(* Logix 5000 Rung export; software revision 16.04 *)

MODULES
   Local : vendor None type None code None
   MVI56E_AFC : vendor None type None code None
END_MODULES

TYPE AFCEProveProcess :   // Prove process output from processor to the module
STRUCT
   Sequencing : AFCEProveSequencing;   // Prover sequencing
   Temperature : REAL;   // Temperature for Single Probe provers. And Inlet Temperature for Dual Probe Provers.
   OutletTemperature : REAL;   // Outlet Temperature for Provers with Dual Probes.
   SwitchBarTemperature : REAL;   // Switch bar temperature
   Pressure : REAL;   // Pressure for Single Probe provers. And Inlet Pressure for Dual Probe Provers.
   OutletPressure : REAL;   // Outlet Pressure for Provers with Dual Probes.
   ProverDensity : REAL;   // Prover density
END_STRUCT
END_TYPE

TYPE AFCEMeterControl :   // Enable/Disable Meter and Streams
STRUCT
   Meter : AFCEMeterControlMeter;   // Control the Meter
   Stream : AFCEMeterControlStream;   // Control the Meter Streams
   ResetAccumulators : AFCEMeterSignals;   // Resets for meter accumulators
END_STRUCT
END_TYPE

TYPE AFCEModbusMasterDataType :   // Modbus master data type
STRUCT
   Bit : BOOL;   // bit type
   Word : BOOL;   // word type (16-bit)
   Long : BOOL;   // long integer (32-bit)
   LongRemote : BOOL;   // long integer (32-bit)
END_STRUCT
END_TYPE

TYPE AFCEProveSequencing :   // AFC prove sequencing tag for phase selection and ball positioning
STRUCT
   Phase : AFCEProvePhaseBitmap;   // AFC phase sequencing
   BallPositionReady : BOOL;   // Ball position: Ready (Udir & Bdir only; fwd leg Bdir)
   BallPositionSealed : BOOL;   // Ball position: Sealed (Udir & Bdir only; fwd leg Bdir)
   BallPositionReadyBwdLeg : BOOL;   // Ball position: Ready bwd leg (Bdir only)
   BallPositionSealedBwdLeg : BOOL;   // Ball position: Sealed bwd leg (Bdir only)
END_STRUCT
END_TYPE

TYPE AFCEMeterLinearLiquidArchiveWrite :   // Write Archive
STRUCT
   Daily : BOOL;   // Set to 1 to write daily archive
   Hourly : BOOL;   // Set to 1 to write hourly archive
END_STRUCT
END_TYPE

TYPE AFCEMeterLinearLiquidProcess :   // Linear Liquid Process Variables
STRUCT
   PulseFrequency : REAL;   // Pulse frequency (Hz)
   Temperature : REAL;   // Temperature
   Pressure : REAL;   // Pressure
   Density : REAL;   // Density
   WaterPercent : REAL;   // Water (%)
   MeterPulses : DINT;   // Meter pulses
END_STRUCT
END_TYPE

TYPE AFCEMeterLinearLiquidAlarm :
STRUCT
   Control : AFCEMeterLinearLiquidAlarmControl;   // Alarm Control
END_STRUCT
END_TYPE

TYPE AFCEUtil :   // Used for internal ladder logic usage. These values must not be changed by user application.
STRUCT
   Flags : AFCEFlag;   // Wallclock update commands
   CycleCounter : INT;   // Reflects current block ID calculated by ladder to be sent to the module
   Buffer : AFCEUtilBuffer;
   Block : AFCEUtilBlock;
END_STRUCT
END_TYPE

TYPE AFCEExtended :
STRUCT
   Trigger : BOOL;
   Data : AFCEExtendedData;
END_STRUCT
END_TYPE

TYPE AFCEModbusGatewayCommand :   // Modbus Gateway Command
STRUCT
   Config : AFCEModbusGatewayConfig;   // Config data to be entered by the user.
   Trigger : BOOL;   // Trigger the Command, when cleared module has responded.
   Data : INT[200];   // Contains modbus data written to the module (write commands)
END_STRUCT
END_TYPE

TYPE AFCEMeterLinearLiqBackPlaneReturn :   // Linear Liquid Meter
STRUCT
   StandardDefault : AFCEMeterLinearLiquidStandardDflt;
   StandardRaw : INT[14];
   Extended : AFCEExtended;
END_STRUCT
END_TYPE

TYPE AFCEMeterStatusStream :
STRUCT
   Active : INT;   // Current Active Stream
   Enabled : AFCEMeterStatusStreamEnabled;   // Enabled Streams
   Configured : AFCEMeterStatusStreamEnabled;   // Configured Streams
   EnableAlarm : AFCEMeterStatusStreamAlarm;   // Enable Alarms
END_STRUCT
END_TYPE

TYPE AFCEProveRunResults :   // Run results of the prove. Copied from the module to the pocessor
STRUCT
   CountAttempted : INT;   // Run count attempted
   CountCompleted : INT;   // Run count completed
   CountSelected : INT;   // Run count selected
   RunsSelected : INT;   // Bit Mapped Runs selected for calculations from completed runs
   NewMeterFactor : REAL;   // New meter factor
   ChangeInMeterFactor : REAL;   // Change in meter factor
END_STRUCT
END_TYPE

TYPE AFCEModbusMasterSwap :   // Modbus master swap words/ swap bytes
STRUCT
   SwapWords : BOOL;   // Swap words
   SwapBytes : BOOL;   // Swap bytes
END_STRUCT
END_TYPE

TYPE AFCEModbusMaster :   // Modbus Master. Port 3 must be configured as modbus master through AFC Manager to use this feature.
STRUCT
   Enable : BOOL;   // Enable the modbus master funcionality
   CommandIndex : INT;   // Selects which command index will be executed
   Command : AFCEModbusMasterCommand[10];   // Each command contains a specific modbus request to be sent out of the port
END_STRUCT
END_TYPE

TYPE AFCEMeterLinearLiquidCalRequestProces :
STRUCT
   PulseFrequency : BOOL;   // Pulse Frequency
   Temperature : BOOL;   // Temperature
   Pressure : BOOL;   // Pressure
   Density : BOOL;   // Density
   WaterContent : BOOL;   // Water Content
END_STRUCT
END_TYPE

TYPE AFCEFlag :   // Flags contains status information updated by ladder and also trigger bits for clock update
STRUCT
   AFCStopped : BOOL;   // Indicates that the module has sent a new input block to be processed by ladder - UPDATED BY LADDER
   AFCInputSequenceNum : INT;   // Meter number (0 -15) associated to blocks 1-16. Used to update "Profile" (meter type and product group.) UPDATED BY LADDER
END_STRUCT
END_TYPE

TYPE AFCEModbusPassThruBitData :   // AFC Modbus Pass-thru Bit Data
STRUCT
   Data : BOOL[2016];   // Contains received data for bit commands
END_STRUCT
END_TYPE

TYPE AFCEUtilBlockInterrupt :
STRUCT
   Now : BOOL;
   ModbusGateway : DINT;
   EnableDisable : BOOL;
   Analysis : DINT;
END_STRUCT
END_TYPE

TYPE AFCEFirmwareVersion :
STRUCT
   Major : SINT;   // Major Version number
   Minor : SINT;   // Minor Version number
   Revision : INT;   // Revision
END_STRUCT
END_TYPE

TYPE AFCEModbusGateway :   // Modbus Gateway
STRUCT
   Command : AFCEModbusGatewayCommand[10];   // Modbus gateway commands - contains setup and modbus data
END_STRUCT
END_TYPE

TYPE AFCEMeterCalRequestActionType :
STRUCT
   ZeroShift : BOOL;   // Zero Shift
   SetZero : BOOL;   // Set Zero
   SetSpan : BOOL;   // Set Span
   SetMid1 : BOOL;   // Set Mid 1
   SetMid2 : BOOL;   // Set Mid 2
   SetMid3 : BOOL;   // Set Mid 3
END_STRUCT
END_TYPE

TYPE AFCEUtilBuffer :   // Buffer
STRUCT
   Input : INT[250];   // Input buffer contains the complete block to be copied from the module
   Output : INT[248];   // Output buffer contains data the complete block to be copied to the module
   Process : INT[240];
   ArchiveDay : INT[98];
   ArchiveHour : INT[98];
   Prove : INT[26];
   Analysis : INT[198];
   MeterEnableDisable : INT[4];
   StreamEnable : INT[48];
   StreamDisable : INT[48];
   StreamSelect : INT[32];
   MeterSignals : INT[32];
   Calibration : INT[36];
END_STRUCT
END_TYPE

TYPE AFCEUtilBlock :
STRUCT
   ProcessInput : INT;
   InterruptPending : AFCEUtilBlockInterrupt;
   InterruptComplete : AFCEUtilBlockInterrupt;
   NonInterruptPending : AFCEUtilBlockNonInterrupt;
   NonInterruptComplete : AFCEUtilBlockNonInterrupt;
END_STRUCT
END_TYPE

TYPE AFCEMeterSignals :   // Meter trigger accumulator and archive resets
STRUCT
   ResetAccumulator1 : BOOL;   // Set to 1 to reset resettable accumulator 1
   ResetAccumulator2 : BOOL;   // Set to 1 to reset resettable accumulator 2
   ResetAccumulator3 : BOOL;   // Set to 1 to reset resettable accumulator 3
   ResetAccumulator4 : BOOL;   // Set to 1 to reset resettable accumulator 4
END_STRUCT
END_TYPE

TYPE AFCEProve :   // Prove
STRUCT
   Process : AFCEProveProcess;   // Process Variables
   Signals : AFCEProveSignals;   // AFC Prove Signals (triggers the proving update)
   Config : AFCEProveConfig;   // AFC Prove Control (configuration settings)
   PulseCounts : AFCEProvePulseCount;   // Pulse counts to be updated at the end of the run/pass
   ConfigInput : AFCEProveInputConfig;   // AFC prover input configuration
   Status : AFCEProveStatus;   // AFC prover status
   ErrorCode : INT;   // Prove error code
   ProveControlsEcho : INT;   // AFC module Echos the state of the Prove Controls
   RequestedMeterEcho : INT;   // AFC module Echos the Meter number requested
   RequestedCurvePointEcho : INT;   // AFC module Echos the requested Curve Point
   RunResults : AFCEProveRunResults;   // Prove and run results
   ProveEnabled : BOOL;   // ON if prove is enabled. This flag is coped from inputbuffer[247]
END_STRUCT
END_TYPE

TYPE AFCEMeterControlStream :
STRUCT
   Selected : SINT;   // Stream to Enable or Disable and/or make active.
   EnableSelected : BOOL;   // Enable the Selected Stream
   DisableSelected : BOOL;   // Disable the Selected Stream
   SetSelectedToActive : BOOL;   // Set Selected to Active Stream
END_STRUCT
END_TYPE

TYPE AFCEProveConfig :   // Controls (configuration settings) associated to the prover
STRUCT
   Enable : AFCEProveConfigEnable;   // Controls at enable
   Accept : AFCEProveConfigAccept;   // Controls at accept
END_STRUCT
END_TYPE

TYPE AFCEWallclock :
STRUCT
   GetAFCTime : BOOL;   // Get current AFC Time
   SetAFCTimeFromPLCTime : BOOL;   // Set AFC time from PLC time. Updates current AFC time
   EnableLocalDateTime : BOOL;   // Enable Local Date Time.
   AFCTime : AFCETime;   // Coordinated Universal Time. Updated by either getting or setting AFC time.
END_STRUCT
END_TYPE

TYPE AFCEMeterCalRequestActionValue :
STRUCT
   ZeroShift : AFCEMeterCalRequestValue;   // Zero Shift
   SetZero : AFCEMeterCalRequestValue;   // Set Zero
   SetSpan : AFCEMeterCalRequestValue;   // Set Span
   SetMid1 : AFCEMeterCalRequestValue;   // Set Mid 1
   SetMid2 : AFCEMeterCalRequestValue;   // Set Mid 2
   SetMid3 : AFCEMeterCalRequestValue;   // Set Mid 3
END_STRUCT
END_TYPE

TYPE AFCEMeterStatus :   // Status
STRUCT
   Meter : AFCEMeterStatusMeter;   // Meter Status
   Stream : AFCEMeterStatusStream;   // Stream Status
END_STRUCT
END_TYPE

TYPE AFCEModbusMasterConfig :   // Modbus master command settings
STRUCT
   Enable : BOOL;   // Set to 1 to enable command (0=disable)
   FunctionType : BOOL;   // Set to 1 to select write command (0=read command)
   RegisterBank : BOOL;   // Set to 1 to select input register (0=holding register)
   DataType : AFCEModbusMasterDataType;   // Select data type format
   SwapOption : AFCEModbusMasterSwap;   // Select byte and word swap (1 = swap, 0 = no swap)
   TypeSwap : INT;   // This value is calculated by ladder logic and must not be modified by user
   SlaveAddress : INT;   // Modbus slave address of remote device
   ModbusAddress : INT;   // Modbus data address on remote slave
   ElementCount : INT;   // Number of data elements (125 words)
   TransactionID : INT;   // Transaction ID. This value is returned to the ReturnedTransaction ID when the response has been received.
END_STRUCT
END_TYPE

TYPE AFCEMeterStatusStreamEnabled :   // Stream Status 1 = Enabled
STRUCT
   Stream1 : BOOL;
   Stream2 : BOOL;
   Stream3 : BOOL;
   Stream4 : BOOL;
   Stream5 : BOOL;
   Stream6 : BOOL;
   Stream7 : BOOL;
   Stream8 : BOOL;
   Stream9 : BOOL;
   Stream10 : BOOL;
   Stream11 : BOOL;
   Stream12 : BOOL;
   Stream13 : BOOL;
   Stream14 : BOOL;
   Stream15 : BOOL;
   Stream16 : BOOL;
END_STRUCT
END_TYPE

TYPE AFCEMeterArchiveFetchError :
STRUCT
   ArchiveSelectionInvalid : BOOL;   // Archive File Selection Invalid
   AgeOutsideSize : BOOL;   // Age Outside Configured File Size
   ArchiveNeverWritten : BOOL;   // Age OK but Archive Record Never Written (new or reconfigured meter)
   Reserverd1 : BOOL;
   Reserverd2 : BOOL;
   Reserverd3 : BOOL;
   Reserverd4 : BOOL;
   Reserverd5 : BOOL;
   Reserverd6 : BOOL;
   Reserverd7 : BOOL;
   Reserverd8 : BOOL;
   Reserverd9 : BOOL;
   Reserverd10 : BOOL;
   Reserverd11 : BOOL;
   Reserverd12 : BOOL;
   Reserverd13 : BOOL;
END_STRUCT
END_TYPE

TYPE AFCEMeterLinearLiquidArchiveDflt :   // Default Configuration
STRUCT
   ClosingTimestamp : DINT;   // Closing Timestamp
   CumulativeActiveStreams : INT;
   CurrentActiveStream : SINT;
   MeterStatus : SINT;
   FlowingPeriod : DINT;
   PeriodDuration : DINT;
   AccumulatorTotalizer : DINT;
   AccumulatorResidue : REAL;
   MeterAlarms : DINT;
   PulseFrequency : REAL;
   Temperature : REAL;
   Pressure : REAL;
   Density : REAL;
   WaterContent : REAL;
   ReferenceDensity : REAL;
   Ctpl : REAL;
   KFactor : REAL;
   MeterFactor : REAL;
   InputPulseCount : DINT;
   ManPulseCountCurrent : DINT;
   MassNRAccumulatorCurrent : REAL;   // Non-resettable
   MassNRAccumulatorOpening : REAL;   // Non-resettable
   Available01 : INT;
   Available02 : INT;
   Available03 : INT;
   Available04 : INT;
   NetNRAccumulatorCurrent : REAL;   // Non-resettable
   NetNRAccumulatorOpening : REAL;   // Non-resettable
   GrossNRAccumulatorCurrent : REAL;   // Non-resettable
   GrossNRAccumulatorOpening : REAL;   // Non-resettable
   GrossStandardNRAccumulatorOpening : REAL;   // Non-resettable
   GrossStandardNRAccumulatorCurrent : REAL;   // Non-resettable
   WaterNRAccumulatorCurrent : REAL;   // Non-resettable
   WaterNRAccumulatorOpening : REAL;   // Non-resettable
   API2540VaporPressureAbsolute : REAL;
   Available05 : INT;
   Available06 : INT;
   UserSpecifiedFlowAverage1 : REAL;
   UserSpecifiedFlowAverage2 : REAL;
   UserSpecifiedFlowAverage3 : REAL;
END_STRUCT
END_TYPE

TYPE AFCEMeterLinearLiquidAlarmControl :   // Linear Liquid Process Alarms
STRUCT
   PulseFrequency : AFCEMeterProcessAlarm;   // Pulse Frequency Alarms
   Temperature : AFCEMeterProcessAlarm;   // Temperature Alarms
   Pressure : AFCEMeterProcessAlarm;   // Pressure Alarms
   Density : AFCEMeterProcessAlarm;   // Density Alarms
   WaterPercent : AFCEMeterProcessAlarm;   // Water Percent Alarms
   MeterPulses : AFCEMeterProcessAlarmFidelity;   // Meter Pulses Alarms
END_STRUCT
END_TYPE

TYPE AFCEMeterLinearLiquidCal :   // Processor Mediated Calibration
STRUCT
   Request : AFCEMeterLinearLiquidCalRequest;   // Calibration Request from module
   Response : AFCEMeterCalResponse;   // Processor Response
END_STRUCT
END_TYPE

TYPE AFCEMeterLinearLiquidArchive :   // Different Liquid Archive
STRUCT
   Write : AFCEMeterLinearLiquidArchiveWrite;
   Fetch : AFCEMeterLinearLiquidArchiveFetch;
END_STRUCT
END_TYPE

TYPE AFCESiteStatus :   // Site status bits - contains general information about the module - not meter specific
STRUCT
   AFCActive : BOOL;   // AFC active
   ChecksumAlarms : BOOL;   // Checkum alarm active
   Reserved2 : BOOL;
   Reserved3 : BOOL;
   PLCHalted : BOOL;   // PLC in program mode or missing
   CfgChanged : BOOL;   // Configuration changed
   Powerup : BOOL;   // Module powered up
   ColdStart : BOOL;   // Module performed cold start (BBRAM initialized)
   ModbusMasterPending : BOOL;   // Modbus Master Poll Pending
   ModbusMasterComplete : BOOL;   // Modbus Master Poll Complete
   ModbusPassThruPending : BOOL;   // Modbus Pass-thru Input Pending
   CalibrationRequest : BOOL;   // Calibration request from module
   ProverEnabled : BOOL;   // Prover Enabled
   Reserved13 : BOOL;
   Reserved14 : BOOL;
   Reserved15 : BOOL;
END_STRUCT
END_TYPE

TYPE AFCEModuleDef :   // Main user defined data type
STRUCT
   ModbusGateway : AFCEModbusGateway;   // Reads and write data between processor and module modbus table
   ModbusMaster : AFCEModbusMaster;   // Setup modbus master commands to be sent to remote slaves (through Port 3)
   ModbusPassThru : AFCEModbusPassThru;   // Modbus pass-thru data
   SiteStatus : AFCESiteStatus;   // Site status
   MeterAlarms : AFCESiteAlarms;   // Meter Alarms
   Prove : AFCEProve;   // Prover
   Wallclock : AFCEWallclock;   // Set clock and get clock information
   Firmware : AFCEFirmwareVersion;   // Firmware information
   Util : AFCEUtil;   // Used by ladder logic
END_STRUCT
END_TYPE

TYPE AFCEModbusGatewayConfig :   // Modbus Ggateway Configuration
STRUCT
   Enable : BOOL;   // Set to 1 to enable modbus gateway command (0=disable)
   StartRegister : DINT;   // Start modbus address
   RegisterCount : INT;   // Word count (200 max)
   FunctionType : BOOL;   // 0 = read command, 1 = write command
   RegisterType : BOOL;   // 0 = holding register, 1 = input register
   SlaveType : BOOL;   // 0 = primary slave, 1 = virtual slave
END_STRUCT
END_TYPE

TYPE AFCEMeterLinearLiquidArchiveFetchT :   // Fetch Archive
STRUCT
   Trigger : BOOL;   // Trigger Archive Fetch
   Age : INT;   // 0 = Current Archive
   Error : AFCEMeterArchiveFetchError;   // Archive Fetch Error
   Default : AFCEMeterLinearLiquidArchiveDflt;   // Default Archive
   Raw : INT[100];   // Raw Archive
END_STRUCT
END_TYPE

TYPE AFCEMeterCalRequestValue :
STRUCT
   Applied : REAL;   // Applied
   Measured : REAL;   // Measured
END_STRUCT
END_TYPE

TYPE AFCEMeterProcessAlarmFidelity :   // Process Alarms
STRUCT
   SetGeneralFail : BOOL;   // Set to indicate General Failure of the Transmitter
   StaleData : BOOL;   // Clear to Indicate new process input data
   Reserved : BOOL;   // Reserved
   SetPulseFidelityAlarm : BOOL;   // Set to indicate Pulse Fidelity Alarm
   SetAutoClearStaleData : BOOL;   // Set to automatically clear stale data
END_STRUCT
END_TYPE

TYPE AFCEUtilBlockNonInterrupt :
STRUCT
   Now : BOOL;
   ModbusMasterCommand : BOOL;
   ModbusMasterResponse : BOOL;
   Archive : DINT;
   Prover : BOOL;
   PassThru : BOOL;
   Calibration : BOOL;
END_STRUCT
END_TYPE

TYPE AFCEMeterLinearLiquid :   // Linear Liquid Meter
STRUCT
   Control : AFCEMeterControl;   // Meter Control
   Status : AFCEMeterStatus;   // Meter Status
   ProcessVariables : AFCEMeterLinearLiquidProcess;   // Input process variables to be transferred to the module
   Alarm : AFCEMeterLinearLiquidAlarm;   // Meter Alarms
   Archive : AFCEMeterLinearLiquidArchive;   // Archive
   Profile : AFCEMeterProfile;   // Module profile (meter type/product group) transfered from the module
   Calibration : AFCEMeterLinearLiquidCal;   // Calibration
   BackPlaneReturn : AFCEMeterLinearLiqBackPlaneReturn;
END_STRUCT
END_TYPE

TYPE AFCEProveConfigAccept :   // Prove controls at accept. If auto-accept is selected must be available at enable
STRUCT
   RequestedInterpolationPoint : INT;   // Requested interpolation point (0 nearest)
   ApplyMFChangeAllStreams : BOOL;   // Apply change in meter factor to all streams
   ApplyMFChangeCurve : BOOL;   // Apply change in meter factor to all curve points
   ApplyNewMF : BOOL;   // CApply new meter factor
END_STRUCT
END_TYPE

TYPE AFCEProvePhaseBitmap :   // AFC prove phase bitmap
STRUCT
   NotSelected : BOOL;   // Not selected
   Active : BOOL;   // Active, not counting
   CountingPast1stSwitch : BOOL;   // Counting past 1st switch for Udir and forward leg for Bdir)
   Past2ndSwitchFwdLeg : BOOL;   // Past 2nd switch forward leg (bidirectional only)
   Past1stSwithRetLeg : BOOL;   // Past 1st switch return leg (bidirectional only)
   RunComplete : BOOL;   // Run complete. past 2nd switch.
END_STRUCT
END_TYPE

TYPE AFCETime :   // AFC time format used for wallclock update.
STRUCT
   Year : DINT;   // Year
   Month : DINT;   // Month
   Day : DINT;   // Day
   Hour : DINT;   // Hour
   Minute : DINT;   // Minute
   second : DINT;   // Seconds
END_STRUCT
END_TYPE

TYPE AFCEProveSignals :   // Contains the proving signals that will trigger specific tasks from the module
STRUCT
   EnableProve : BOOL;   // Enables the prove
   AcceptProve : BOOL;   // Accepts the prove
   RejectProve : BOOL;   // Reject the prove
   RunStart : BOOL;   // Starts the run
   RunComplete : BOOL;   // Flags that the run is complete
   RunCancel : BOOL;   // Cancels the run
   RunDelete : BOOL;   // Deletes the run
   PassComplete : BOOL;   // Flag that the pass is complete
   PauseProve : BOOL;   // Pauses the Proving Process
   AbortProve : BOOL;   // Aborts the prove
END_STRUCT
END_TYPE

TYPE AFCEMeterProfile :   // Meter configuration profile
STRUCT
   MeterType : BOOL;   // 0=Differential, 1=Linear
   ProductGroup : BOOL;   // 0=Gas, 1=Liquid
   PrimaryInput : BOOL;   // For differential, 0=Differential Pressure 1=Flow Rate. For Linear, 0=Pulse Count 1=Pulse Frequency
   AOIMismatch : BOOL;   // AOI Meter type does not match module for meter number
END_STRUCT
END_TYPE

TYPE AFCEMeterStatusStreamAlarm :   // Stream Alarms
STRUCT
   StreamOutOfRange : BOOL;   // Requested Stream Number Out of Range
   StreamNotConfigured : BOOL;   // Requested Stream not Configured
   StreamNotEnabled : BOOL;   // Requested Stream not Enabled
   EventLogFull : BOOL;   // Event Log Full, Action not Performed
END_STRUCT
END_TYPE

TYPE AFCEModbusPassThru :   // AFC Modbus Pass-thru
STRUCT
   Enable : BOOL;   // Set to 1 to enable pass-thru functionality (requires AFC Manager setting)
   MessagePresent : BOOL;   // Message present in the response block
   GetMessage : BOOL;   // Get the pass-thru message. When the bit is cleared the message has been transferred to the PLC.
   FunctionBitWrite : BOOL;   // Function bit write
   OverflowError : BOOL;   // Overflow error flag
   ModbusAddress : INT;   // Destination modbus address
   RegisterCount : INT;   // Number of elements associated to command
   ReadDataWord : INT[125];   // Contains received data for word commands
   ReadDataBit : AFCEModbusPassThruBitData;   // Contains received data for bit commands
END_STRUCT
END_TYPE

TYPE AFCEProveInputConfig :   // Prove input block results - prover configuration
STRUCT
   Type : INT;   // Prover type
   Options : INT;   // Prover options
   RunsPerProveTotal : INT;   // Total runs per prove
   RunsPerProveSelected : INT;   // Selected runs per prove
   MaxRunsBeforeAbort : INT;   // Max total runs before abort
   ShortPassesPerRun : INT;   // Short passes per run if bidir = 2 , else 0
END_STRUCT
END_TYPE

TYPE AFCEMeterLinearLiquidArchiveFetch :
STRUCT
   Daily : AFCEMeterLinearLiquidArchiveFetchT;
   Hourly : AFCEMeterLinearLiquidArchiveFetchT;
END_STRUCT
END_TYPE

TYPE AFCEMeterLinearLiquidStandardDflt :   // Linear Liquid Meter Default Standard Data
STRUCT
   Meter_Alarms : DINT;   // Meter alarms
   NR_Acc_Net_Totalizer : DINT;   // Non-resettable accumulator, net, totalizer (m3)
   NR_Acc_Net_Residue : REAL;   // Non-resettable accumulator, net, residue (m3)
   FlowRate_Net : REAL;   // Flow rate, net (m3/h)
   NR_Acc_Gross_Totalizer : DINT;   // Non-resettable accumulator, gross / indicated, totalizer (m3)
   NR_Acc_GrossStandard_Totalizer : DINT;   // Non-resettable accumulator, gross standard, totalizer (m3)
   NR_Acc_Mass_Totalizer : DINT;   // Non-resettable accumulator, mass, totalizer (kg)
END_STRUCT
END_TYPE

TYPE AFCEProveStatus :   // Status of the prove (returned from the module to the processor)
STRUCT
   ProveAccepted : BOOL;   // Prove was accepted
   MeterFactorApplied : BOOL;   // Meter factor was applied
   MFAppliedToCurve : BOOL;   // Meter factor was applied to all points in the curve
   MFAppliedToStreams : BOOL;   // Meter factor was applied to all streams
   ProveRejectedByCommand : BOOL;   // Prove was rejected by command
   ProveRejectedNoRuns : BOOL;   // Prove was rejected - empty prove (no runs)
   ProveRejectedDivideBy0 : BOOL;   // Prove was rejected - divide by 0
   ProveEnabled : BOOL;   // Prove is enabled
   ProvingRunInProgress : BOOL;   // Proving run is in progress
   ProveRejectedAbort : BOOL;   // Prove rejected: abort
   ProvePaused : BOOL;   // Prove is paused
   RunCancelled : BOOL;   // Run Is cancelled
   RunTimedOut : BOOL;   // Run timed out
END_STRUCT
END_TYPE

TYPE AFCEMeterProcessAlarm :   // Process Alarms
STRUCT
   SetGeneralFail : BOOL;   // Set to indicate General Failure of the Transmitter
   StaleData : BOOL;   // Clear to Indicate new process input data
   SetLowThreshold : BOOL;   // Set to indicate Lower Range Limit Exceeded
   SetHighThreshold : BOOL;   // Set to indicate Upper Range Limit Exceeded
   SetAutoClearStaleData : BOOL;   // Set to automatically clear stale data
END_STRUCT
END_TYPE

TYPE AFCEProveConfigEnable :   // Prove controls at enable
STRUCT
   MeterNumber : INT;   // Meter number requested (1-16)
   AutoAcceptProve : BOOL;   // Auto-accept the prove
   AutoContinueProve : BOOL;   // Auto-continue the prove
END_STRUCT
END_TYPE

TYPE AFCEMeterStatusMeter :   // Meter Status
STRUCT
   Enabled : BOOL;   // Meter Enable Status, 1=enabled
   EnableAlarm : BOOL;   // If set either: 1. The meter is not configured. 2. The event log is full, the action was not performed.
END_STRUCT
END_TYPE

TYPE AFCEMeterControlMeter :   // Enable and Disable Meter
STRUCT
   Enable : BOOL;   // Enable the Meter
   Disable : BOOL;   // Disable the Meter
END_STRUCT
END_TYPE

TYPE AFCEModbusMasterCommand :   // Modbus Master Command
STRUCT
   Config : AFCEModbusMasterConfig;   // Modbus Master Configuration
   ErrorCode : INT;   // Error Code associated to Modbus Master Command
   Pending : BOOL;   // Pending Modbus Master Command - waiting for Modbus Response
   ReturnedTransactionID : DINT;   // Changes to Config.TransactionID value when response has returned.
   Data : INT[100];   // Read or Write Data
END_STRUCT
END_TYPE

TYPE AFCEProvePulseCount :   // Values to be supplied at the end of the pass/run
STRUCT
   Meter : DINT;   // Meter pulse count
   MasterMeter : DINT;   // Master meter pulse count
END_STRUCT
END_TYPE

TYPE AFCEMeterCalResponse :
STRUCT
   Trigger : BOOL;   // Send Error Code and Values to module to be recorded
   ErrorCode : SINT;   // Error Code to send. 0-4 allowed. 0=No error. 1-4=User defined.
   Value : AFCEMeterCalRequestValue;   // Value to Send
   Count : DINT;   // Number of calibration responses
END_STRUCT
END_TYPE

TYPE AFCEExtendedData :
STRUCT
   Raw : INT[64];
END_STRUCT
END_TYPE

TYPE AFCEMeterLinearLiquidCalRequest :
STRUCT
   ProcessVariable : AFCEMeterLinearLiquidCalRequestProces;   // Process Variable
   ActionType : AFCEMeterCalRequestActionType;   // Action Type
   Value : AFCEMeterCalRequestActionValue;   // Value
   Count : DINT;   // Number of calibration requests
END_STRUCT
END_TYPE

TYPE AFCESiteAlarms :   // Indicates if a meter has any alarms
STRUCT
   Meter1 : BOOL;   // Meter in alarm
   Meter2 : BOOL;   // Meter in alarm
   Meter3 : BOOL;   // Meter in alarm
   Meter4 : BOOL;   // Meter in alarm
   Meter5 : BOOL;   // Meter in alarm
   Meter6 : BOOL;   // Meter in alarm
   Meter7 : BOOL;   // Meter in alarm
   Meter8 : BOOL;   // Meter in alarm
   Meter9 : BOOL;   // Meter in alarm
   Meter10 : BOOL;   // Meter in alarm
   Meter11 : BOOL;   // Meter in alarm
   Meter12 : BOOL;   // Meter in alarm
   Meter13 : BOOL;   // Meter in alarm
   Meter14 : BOOL;   // Meter in alarm
   Meter15 : BOOL;   // Meter in alarm
   Meter16 : BOOL;   // Meter in alarm
END_STRUCT
END_TYPE

ADD_ON_INSTRUCTION AOI56EAFCMeterLinearLiquid   (* revision 1.7, vendor ProSoft Technology Inc., ExecutePrescan *)
// Add-On instruction for the MVI56E-AFC.
// Linear Liquid Meter
// Revision note:
// Corrected/Reverted ProcessInputBlockID Tag Data Type from INT to DINT.
// Help:
// v1.3: Addition of default process input backplane return data mapping.
// v1.4: Made correlation changes between the Module Archive Default UDTs and the AOI Archive Default UDTs.
// v1.5:  Made changes to the ModbusGatewayConfig UDT StartRegister Tag Data Type from INT to DINT
// and Modified ProcessInputBlockID Tag Data Type from DINT to INT.
// v1.6:  Updated Tags names AFCMeterXXYYYYYY.BackPlaneReturn.ProcessInputs to
// AFCMeterXXYYYYYY.BackPlaneReturn.Standard and
// AFCMeterXXYYYYYY.BackPlaneReturn.ComponentAnalysis
//  to AFCMeterXXYYYYYY.BackPlaneReturn.Extended.
// v1.7:  Corrected/Reverted ProcessInputBlockID Tag Data Type from INT to DINT.
VAR_IN_OUT
   ConnectionInput : INT[250]; {required}
   AFC : AFCEModuleDef; {required}
   AFCMeter : AFCEMeterLinearLiquid; {required}
END_VAR
VAR_INPUT
   MeterNumber : SINT; {required}   // Meter Number Set to a number between 1 and 16
END_VAR
VAR
   StreamSelectedShift : DINT;
   StreamSelectBuffer : INT;
   EnabledStatusBuffer : INT;
   StreamSelectBlockID : DINT;
   StreamNumberShift : DINT;
   StreamErrorBuffer : DINT;
   StreamEnableBlockID : DINT;
   StreamEnableBitPosition : DINT;
   StreamDisableBlockID : DINT;
   ResetOnce : BOOL;
   ProfileBuffer : SINT[2];
   ProcessInputBlockID : DINT;
   AnalysisGroupBitPosition : INT;
   AnalysisErrorBuffer : INT;
   ProcessAlarmShifter : DINT;
   ProcessAlarmHolder : DINT;
   ProcessAlarmBuffer : DINT;
   MeterSignaltBlockID : DINT;
   MeterNumberShift : DINT;
   MeterNumberBitPostition : DINT;
   Inputbuffer : INT[250];
   CalibrationMeterNumberBuffer : DINT;
   CalibrationMediationPending : BOOL;
   CalibrationInputScalingIndex : DINT;
   CalibrationHandleBuffer : DINT;
   ArchiveStream : DINT;
   ArchiveMeterStatusRaw : DINT;
   ArchiveMeterStatusActiveStream : DINT;
   ArchiveCompleteBitCheck : DINT;
   ArchiveBlockID : DINT;
   AnalysisGroupShift : DINT;
   AnalysisCompleteBitCheck : DINT;
   AnalysisBufferOffset : DINT;
   AFCStopped : BOOL;
   AFCInputDataAvailable : BOOL;
   AnalysisBlockID : DINT;
END_VAR

ROUTINE Logic   (* ladder *)
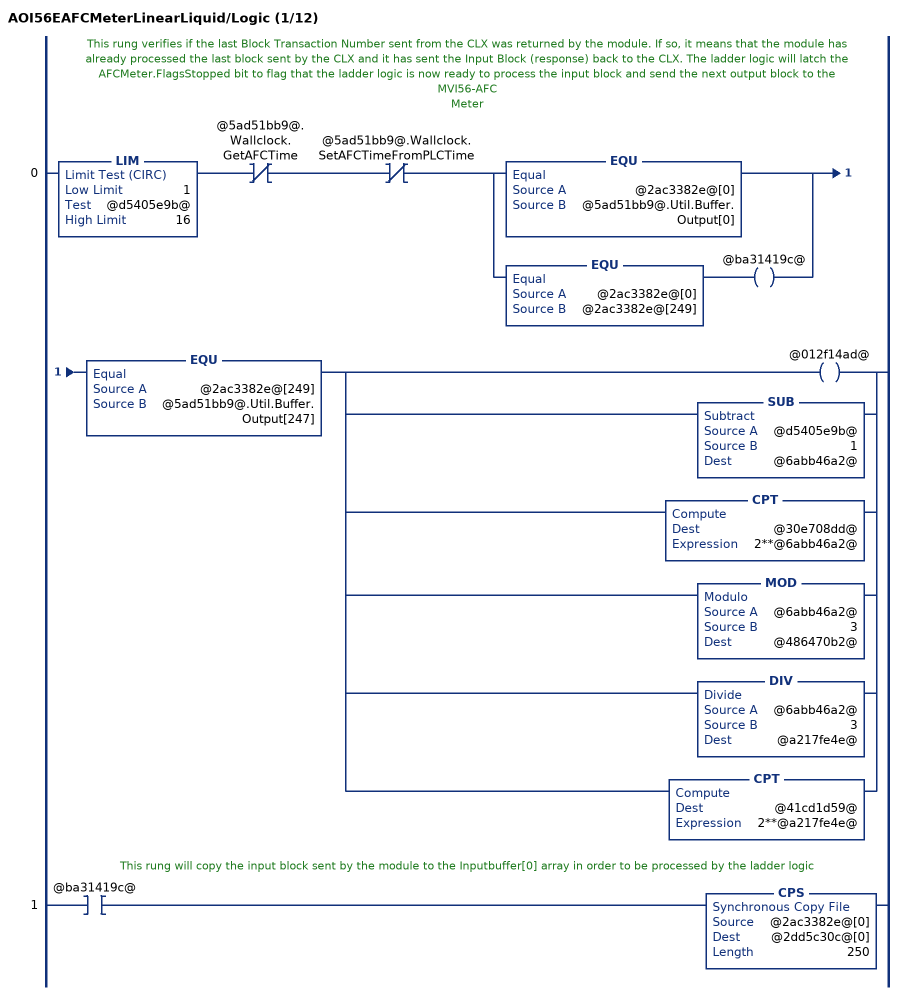
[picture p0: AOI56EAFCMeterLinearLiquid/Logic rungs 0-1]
   // This rung verifies if the last Block Transaction Number sent from the CLX was returned by the module. If so, it means that the module has already processed the last block sent by the CLX and it has sent the Input Block (response) back to the CLX. The ladder logic will latch the AFCMeter.FlagsStopped bit to flag that the ladder logic is now ready to process the input block and send the next output block to the MVI56-AFC
   // Meter
   0: LIM(1,@d5405e9b@,16)XIO(@5ad51bb9@.Wallclock.GetAFCTime)XIO(@5ad51bb9@.Wallclock.SetAFCTimeFromPLCTime)[EQU(@2ac3382e@[0],@5ad51bb9@.Util.Buffer.Output[0]) ,EQU(@2ac3382e@[0],@2ac3382e@[249]) OTE(@ba31419c@) ]EQU(@2ac3382e@[249],@5ad51bb9@.Util.Buffer.Output[247])[OTE(@012f14ad@) ,SUB(@d5405e9b@,1,@6abb46a2@) ,CPT(@30e708dd@,2**@6abb46a2@) ,MOD(@6abb46a2@,3,@486470b2@) ,DIV(@6abb46a2@,3,@a217fe4e@) ,CPT(@41cd1d59@,2**@a217fe4e@) ];
   // This rung will copy the input block sent by the module to the Inputbuffer[0] array in order to be processed by the ladder logic
   1: XIC(@ba31419c@)CPS(@2ac3382e@[0],@2dd5c30c@[0],250);
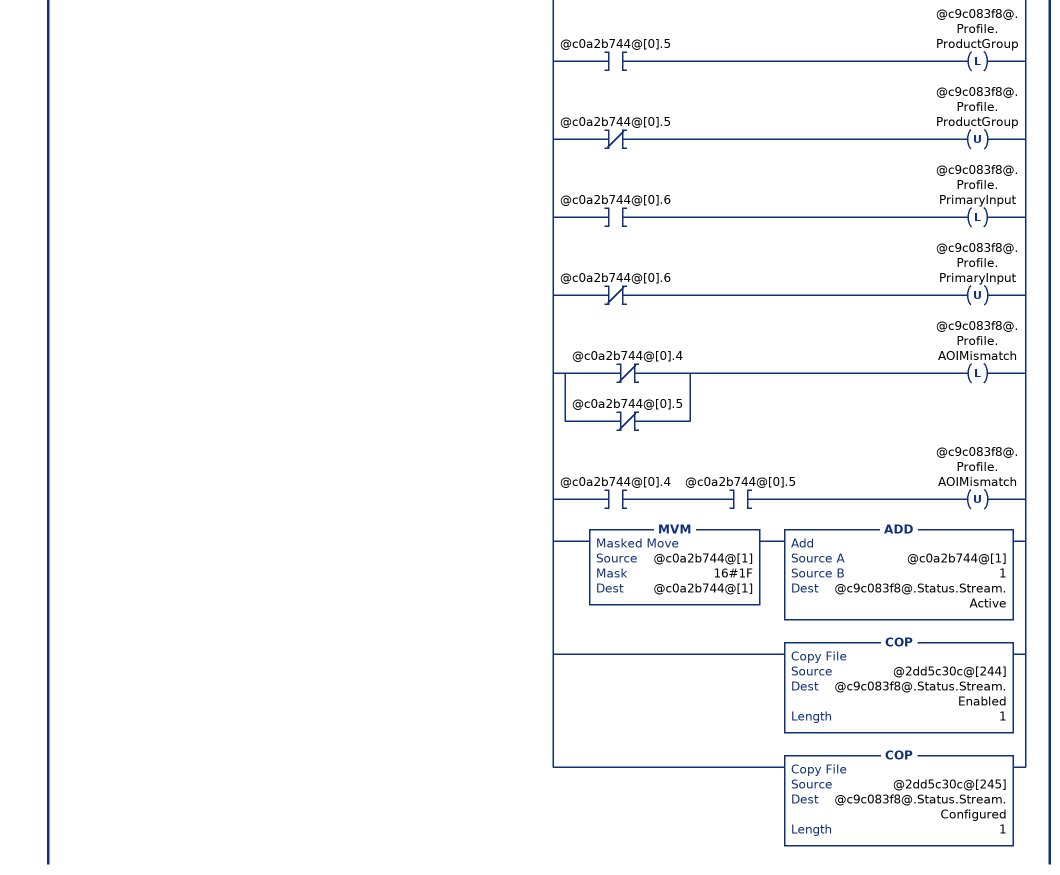
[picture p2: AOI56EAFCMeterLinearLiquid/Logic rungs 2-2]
   // Read process input backplane return and
   // meter profile (when block ID matches meter number).
   2: XIC(@ba31419c@)LIM(1,@2dd5c30c@[0],16)[COP(@2dd5c30c@[3+@6abb46a2@*15],@c9c083f8@.BackPlaneReturn.StandardRaw[0],14) ,COP(@c9c083f8@.BackPlaneReturn.StandardRaw[0],@c9c083f8@.BackPlaneReturn.StandardDefault,1) ,COP(@2dd5c30c@[247],@5ad51bb9@.SiteStatus,1) ,COP(@2dd5c30c@[248],@5ad51bb9@.MeterAlarms,1) ,EQU(@2dd5c30c@[0],@d5405e9b@) [COP(@2dd5c30c@[243],@c0a2b744@[0],2) ,[XIC(@c0a2b744@[0].0) OTL(@c9c083f8@.Status.Meter.EnableAlarm) ,XIO(@c0a2b744@[0].0) OTU(@c9c083f8@.Status.Meter.EnableAlarm) ] ,[XIC(@c0a2b744@[0].1) OTL(@c9c083f8@.Status.Meter.Enabled) ,XIO(@c0a2b744@[0].1) OTU(@c9c083f8@.Status.Meter.Enabled) ] ,[[XIC(@c0a2b744@[0].4) OTL(@c9c083f8@.Profile.MeterType) ,XIO(@c0a2b744@[0].4) OTU(@c9c083f8@.Profile.MeterType) ] ,[XIC(@c0a2b744@[0].5) OTL(@c9c083f8@.Profile.ProductGroup) ,XIO(@c0a2b744@[0].5) OTU(@c9c083f8@.Profile.ProductGroup) ] ,[XIC(@c0a2b744@[0].6) OTL(@c9c083f8@.Profile.PrimaryInput) ,XIO(@c0a2b744@[0].6) OTU(@c9c083f8@.Profile.PrimaryInput) ] ] ,[[XIO(@c0a2b744@[0].4) ,XIO(@c0a2b744@[0].5) ] OTL(@c9c083f8@.Profile.AOIMismatch) ,XIC(@c0a2b744@[0].4) XIC(@c0a2b744@[0].5) OTU(@c9c083f8@.Profile.AOIMismatch) ] ,MVM(@c0a2b744@[1],16#1F,@c0a2b744@[1]) ADD(@c0a2b744@[1],1,@c9c083f8@.Status.Stream.Active) ,COP(@2dd5c30c@[244],@c9c083f8@.Status.Stream.Enabled,1) ,COP(@2dd5c30c@[245],@c9c083f8@.Status.Stream.Configured,1) ] ];
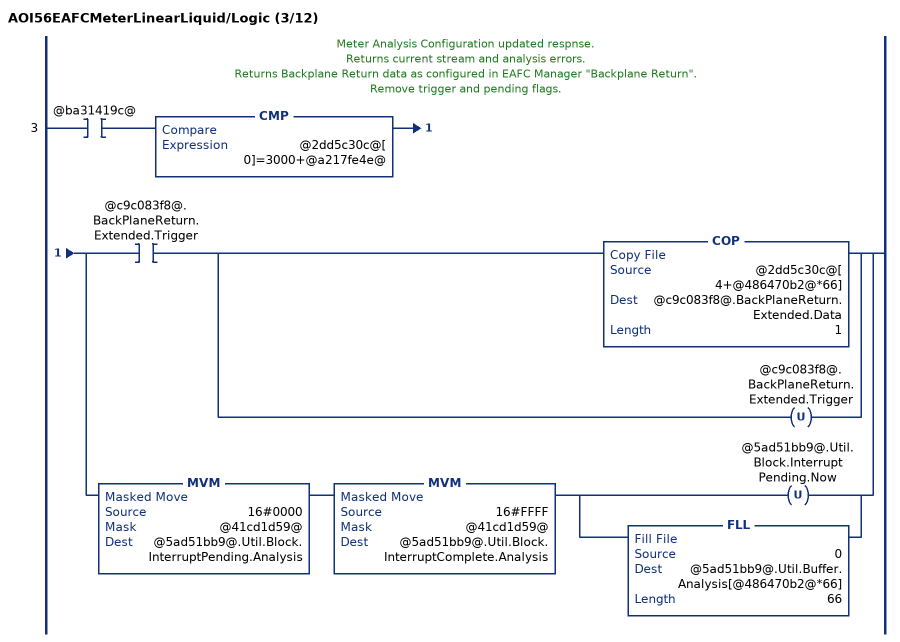
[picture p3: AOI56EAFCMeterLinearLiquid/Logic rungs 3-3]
   // Meter Analysis Configuration updated respnse.
   // Returns current stream and analysis errors.
   // Returns Backplane Return data as configured in EAFC Manager "Backplane Return".
   // Remove trigger and pending flags.
   3: XIC(@ba31419c@)CMP(@2dd5c30c@[0]=3000+@a217fe4e@)[XIC(@c9c083f8@.BackPlaneReturn.Extended.Trigger) [COP(@2dd5c30c@[4+@486470b2@*66],@c9c083f8@.BackPlaneReturn.Extended.Data,1) ,OTU(@c9c083f8@.BackPlaneReturn.Extended.Trigger) ] ,MVM(16#0000,@41cd1d59@,@5ad51bb9@.Util.Block.InterruptPending.Analysis) MVM(16#FFFF,@41cd1d59@,@5ad51bb9@.Util.Block.InterruptComplete.Analysis) [OTU(@5ad51bb9@.Util.Block.InterruptPending.Now) ,FLL(0,@5ad51bb9@.Util.Buffer.Analysis[@486470b2@*66],66) ] ];
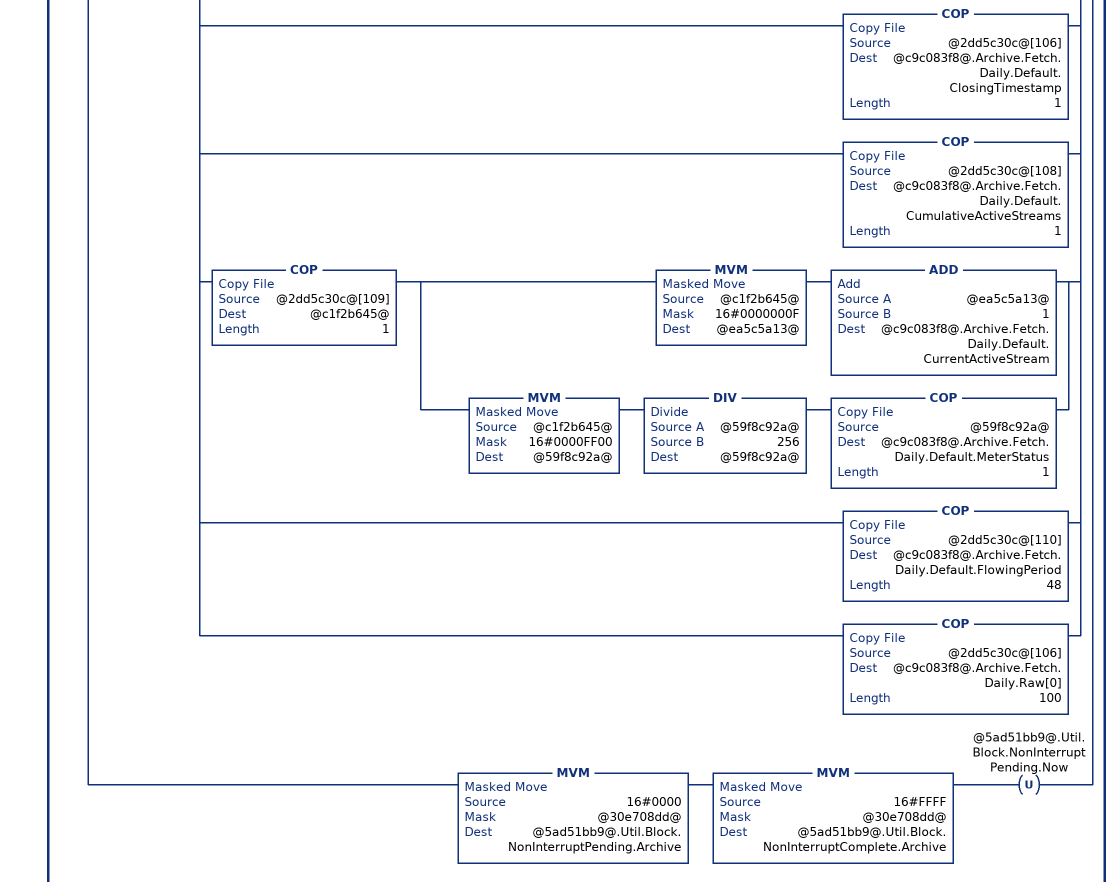
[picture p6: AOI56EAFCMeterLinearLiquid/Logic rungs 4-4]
   // Archive Fetch to default and raw UDT's.
   // Get archive alarms.
   // Remove trigger and pending flags.
   4: XIC(@ba31419c@)CMP(@2dd5c30c@[0]=6000+@6abb46a2@)[XIC(@c9c083f8@.Archive.Fetch.Hourly.Trigger) [OTU(@c9c083f8@.Archive.Fetch.Hourly.Trigger) ,[[XIC(@2dd5c30c@[3].0) OTL(@c9c083f8@.Archive.Fetch.Hourly.Error.ArchiveSelectionInvalid) ,XIO(@2dd5c30c@[3].0) OTU(@c9c083f8@.Archive.Fetch.Hourly.Error.ArchiveSelectionInvalid) ] ,[XIC(@2dd5c30c@[3].1) OTL(@c9c083f8@.Archive.Fetch.Hourly.Error.AgeOutsideSize) ,XIO(@2dd5c30c@[3].1) OTU(@c9c083f8@.Archive.Fetch.Hourly.Error.AgeOutsideSize) ] ,[XIC(@2dd5c30c@[3].2) OTL(@c9c083f8@.Archive.Fetch.Hourly.Error.ArchiveNeverWritten) ,XIO(@2dd5c30c@[3].2) OTU(@c9c083f8@.Archive.Fetch.Hourly.Error.ArchiveNeverWritten) ] ] ,COP(@2dd5c30c@[4],@c9c083f8@.Archive.Fetch.Hourly.Default.ClosingTimestamp,1) ,COP(@2dd5c30c@[6],@c9c083f8@.Archive.Fetch.Hourly.Default.CumulativeActiveStreams,1) ,COP(@2dd5c30c@[7],@c1f2b645@,1) [MVM(@c1f2b645@,16#0000000F,@ea5c5a13@) ADD(@ea5c5a13@,1,@c9c083f8@.Archive.Fetch.Hourly.Default.CurrentActiveStream) ,MVM(@c1f2b645@,16#0000FF00,@59f8c92a@) DIV(@59f8c92a@,256,@59f8c92a@) COP(@59f8c92a@,@c9c083f8@.Archive.Fetch.Hourly.Default.MeterStatus,1) ] ,COP(@2dd5c30c@[8],@c9c083f8@.Archive.Fetch.Hourly.Default.FlowingPeriod,48) ,COP(@2dd5c30c@[4],@c9c083f8@.Archive.Fetch.Hourly.Raw[0],100) ] ,XIC(@c9c083f8@.Archive.Fetch.Daily.Trigger) [OTU(@c9c083f8@.Archive.Fetch.Daily.Trigger) ,[[XIC(@2dd5c30c@[105].0) OTL(@c9c083f8@.Archive.Fetch.Daily.Error.ArchiveSelectionInvalid) ,XIO(@2dd5c30c@[105].0) OTU(@c9c083f8@.Archive.Fetch.Daily.Error.ArchiveSelectionInvalid) ] ,[XIC(@2dd5c30c@[105].1) OTL(@c9c083f8@.Archive.Fetch.Daily.Error.AgeOutsideSize) ,XIO(@2dd5c30c@[105].1) OTU(@c9c083f8@.Archive.Fetch.Daily.Error.AgeOutsideSize) ] ,[XIC(@2dd5c30c@[105].2) OTL(@c9c083f8@.Archive.Fetch.Daily.Error.ArchiveNeverWritten) ,XIO(@2dd5c30c@[105].2) OTU(@c9c083f8@.Archive.Fetch.Daily.Error.ArchiveNeverWritten) ] ] ,COP(@2dd5c30c@[106],@c9c083f8@.Archive.Fetch.Daily.Default.ClosingTimestamp,1) ,COP(@2dd5c30c@[108],@c9c083f8@.Archive.Fetch.Daily.Default.CumulativeActiveStreams,1) ,COP(@2dd5c30c@[109],@c1f2b645@,1) [MVM(@c1f2b645@,16#0000000F,@ea5c5a13@) ADD(@ea5c5a13@,1,@c9c083f8@.Archive.Fetch.Daily.Default.CurrentActiveStream) ,MVM(@c1f2b645@,16#0000FF00,@59f8c92a@) DIV(@59f8c92a@,256,@59f8c92a@) COP(@59f8c92a@,@c9c083f8@.Archive.Fetch.Daily.Default.MeterStatus,1) ] ,COP(@2dd5c30c@[110],@c9c083f8@.Archive.Fetch.Daily.Default.FlowingPeriod,48) ,COP(@2dd5c30c@[106],@c9c083f8@.Archive.Fetch.Daily.Raw[0],100) ] ,MVM(16#0000,@30e708dd@,@5ad51bb9@.Util.Block.NonInterruptPending.Archive) MVM(16#FFFF,@30e708dd@,@5ad51bb9@.Util.Block.NonInterruptComplete.Archive) OTU(@5ad51bb9@.Util.Block.NonInterruptPending.Now) ];
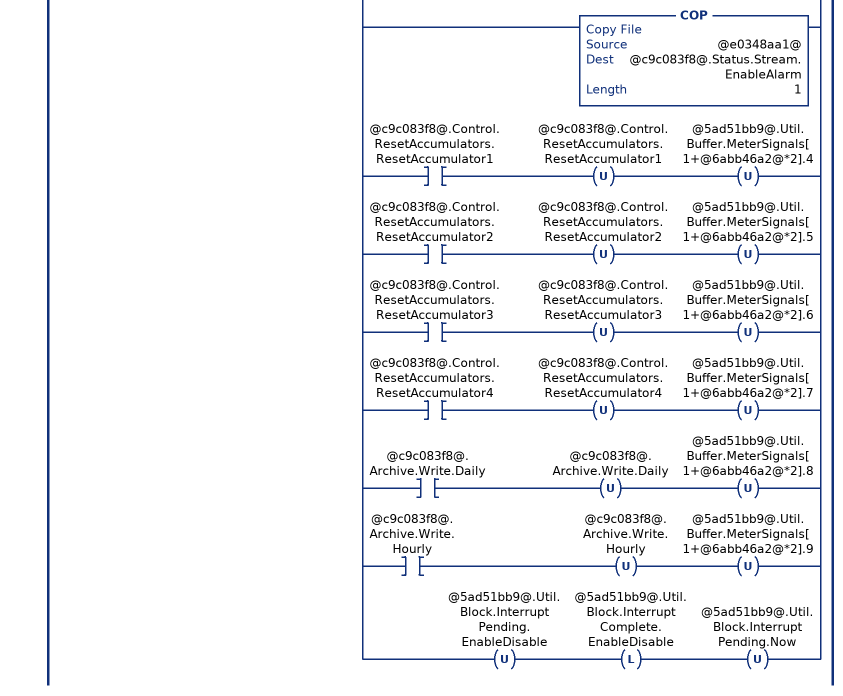
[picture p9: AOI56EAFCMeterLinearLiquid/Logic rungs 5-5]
   // Meter status and stream status.
   // Remove trigger and pending flags.
   5: XIC(@ba31419c@)EQU(@2dd5c30c@[0],7000)[[MVM(@2dd5c30c@[3],@30e708dd@,@a897f87c@) ,[NEQ(@a897f87c@,0) OTL(@c9c083f8@.Status.Meter.Enabled) ,EQU(@a897f87c@,0) OTU(@c9c083f8@.Status.Meter.Enabled) ] ,OTU(@c9c083f8@.Control.Meter.Enable) MVM(16#0000,@30e708dd@,@5ad51bb9@.Util.Buffer.MeterEnableDisable[1]) ,OTU(@c9c083f8@.Control.Meter.Disable) MVM(16#0000,@30e708dd@,@5ad51bb9@.Util.Buffer.MeterEnableDisable[3]) ] ,[XIC(@c9c083f8@.Control.Stream.EnableSelected) [COP(@2dd5c30c@[7+@6abb46a2@*3],@c9c083f8@.Status.Stream.Enabled,1) ,COP(@2dd5c30c@[8+@6abb46a2@*3],@c9c083f8@.Status.Stream.Configured,1) ,OTU(@c9c083f8@.Control.Stream.EnableSelected) OTU(@c9c083f8@.Control.Stream.DisableSelected) ] ,XIC(@c9c083f8@.Control.Stream.DisableSelected) [COP(@2dd5c30c@[55+@6abb46a2@*3],@c9c083f8@.Status.Stream.Enabled,1) ,COP(@2dd5c30c@[56+@6abb46a2@*3],@c9c083f8@.Status.Stream.Configured,1) ,OTU(@c9c083f8@.Control.Stream.EnableSelected) OTU(@c9c083f8@.Control.Stream.DisableSelected) ] ] ,[OTU(@c9c083f8@.Control.Stream.SetSelectedToActive) ,COP(@2dd5c30c@[103+@6abb46a2@*2],@1d93410d@,1) ,[XIC(@1d93410d@.8) OTL(@e0348aa1@.0) ,XIO(@1d93410d@.8) OTU(@e0348aa1@.0) ] ,[XIC(@1d93410d@.9) OTL(@e0348aa1@.1) ,XIO(@1d93410d@.9) OTU(@e0348aa1@.1) ] ,[XIC(@1d93410d@.10) OTL(@e0348aa1@.2) ,XIO(@1d93410d@.10) OTU(@e0348aa1@.2) ] ,[XIC(@1d93410d@.11) OTL(@e0348aa1@.3) ,XIO(@1d93410d@.11) OTU(@e0348aa1@.3) ] ,MVM(@1d93410d@,16#000F,@4a4a3092@) ADD(@4a4a3092@,1,@c9c083f8@.Status.Stream.Active) ,COP(@e0348aa1@,@c9c083f8@.Status.Stream.EnableAlarm,1) ] ,[XIC(@c9c083f8@.Control.ResetAccumulators.ResetAccumulator1) OTU(@c9c083f8@.Control.ResetAccumulators.ResetAccumulator1) OTU(@5ad51bb9@.Util.Buffer.MeterSignals[1+@6abb46a2@*2].4) ,XIC(@c9c083f8@.Control.ResetAccumulators.ResetAccumulator2) OTU(@c9c083f8@.Control.ResetAccumulators.ResetAccumulator2) OTU(@5ad51bb9@.Util.Buffer.MeterSignals[1+@6abb46a2@*2].5) ,XIC(@c9c083f8@.Control.ResetAccumulators.ResetAccumulator3) OTU(@c9c083f8@.Control.ResetAccumulators.ResetAccumulator3) OTU(@5ad51bb9@.Util.Buffer.MeterSignals[1+@6abb46a2@*2].6) ,XIC(@c9c083f8@.Control.ResetAccumulators.ResetAccumulator4) OTU(@c9c083f8@.Control.ResetAccumulators.ResetAccumulator4) OTU(@5ad51bb9@.Util.Buffer.MeterSignals[1+@6abb46a2@*2].7) ,XIC(@c9c083f8@.Archive.Write.Daily) OTU(@c9c083f8@.Archive.Write.Daily) OTU(@5ad51bb9@.Util.Buffer.MeterSignals[1+@6abb46a2@*2].8) ,XIC(@c9c083f8@.Archive.Write.Hourly) OTU(@c9c083f8@.Archive.Write.Hourly) OTU(@5ad51bb9@.Util.Buffer.MeterSignals[1+@6abb46a2@*2].9) ] ,OTU(@5ad51bb9@.Util.Block.InterruptPending.EnableDisable) OTL(@5ad51bb9@.Util.Block.InterruptComplete.EnableDisable) OTU(@5ad51bb9@.Util.Block.InterruptPending.Now) ];
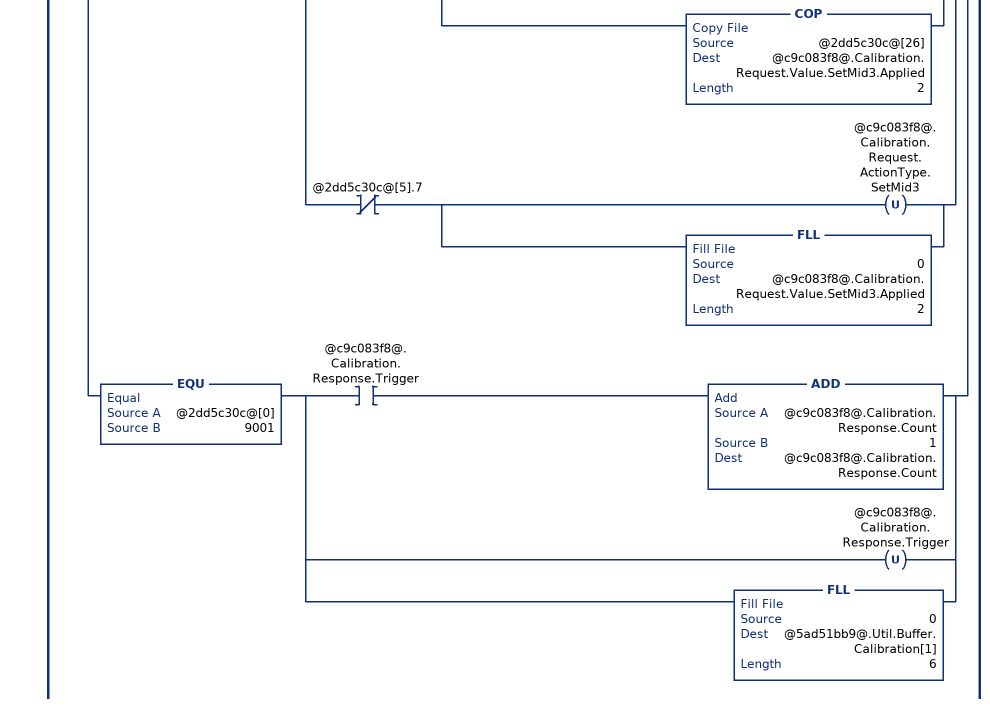
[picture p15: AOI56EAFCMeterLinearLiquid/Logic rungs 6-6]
   // Meter transmitter calibration.
   6: XIC(@ba31419c@)[EQU(@2dd5c30c@[0],9000) ,EQU(@2dd5c30c@[0],9001) ][MVM(@2dd5c30c@[3],16#0F00,@db859ddf@) ,DIV(@db859ddf@,16#100,@db859ddf@) ]EQU(@db859ddf@,@6abb46a2@)XIO(@2dd5c30c@[3].14)[EQU(@2dd5c30c@[0],9000) [XIO(@88c34d46@) ADD(@c9c083f8@.Calibration.Request.Count,1,@c9c083f8@.Calibration.Request.Count) ,OTL(@88c34d46@) [COP(@2dd5c30c@[3],@186447d0@,1) ,MVM(@186447d0@,16#000F,@56e7eb71@) ] ,[EQU(@56e7eb71@,0) [OTL(@c9c083f8@.Calibration.Request.ProcessVariable.PulseFrequency) ,OTU(@c9c083f8@.Calibration.Request.ProcessVariable.Temperature) ,OTU(@c9c083f8@.Calibration.Request.ProcessVariable.Pressure) ,OTU(@c9c083f8@.Calibration.Request.ProcessVariable.Density) ,OTU(@c9c083f8@.Calibration.Request.ProcessVariable.WaterContent) ] ,EQU(@56e7eb71@,1) [OTL(@c9c083f8@.Calibration.Request.ProcessVariable.Temperature) ,OTU(@c9c083f8@.Calibration.Request.ProcessVariable.PulseFrequency) ,OTU(@c9c083f8@.Calibration.Request.ProcessVariable.Pressure) ,OTU(@c9c083f8@.Calibration.Request.ProcessVariable.Density) ,OTU(@c9c083f8@.Calibration.Request.ProcessVariable.WaterContent) ] ,EQU(@56e7eb71@,2) [OTL(@c9c083f8@.Calibration.Request.ProcessVariable.Pressure) ,OTU(@c9c083f8@.Calibration.Request.ProcessVariable.PulseFrequency) ,OTU(@c9c083f8@.Calibration.Request.ProcessVariable.Temperature) ,OTU(@c9c083f8@.Calibration.Request.ProcessVariable.Density) ,OTU(@c9c083f8@.Calibration.Request.ProcessVariable.WaterContent) ] ,EQU(@56e7eb71@,3) [OTL(@c9c083f8@.Calibration.Request.ProcessVariable.Density) ,OTU(@c9c083f8@.Calibration.Request.ProcessVariable.PulseFrequency) ,OTU(@c9c083f8@.Calibration.Request.ProcessVariable.Temperature) ,OTU(@c9c083f8@.Calibration.Request.ProcessVariable.Pressure) ,OTU(@c9c083f8@.Calibration.Request.ProcessVariable.WaterContent) ] ,EQU(@56e7eb71@,4) [OTL(@c9c083f8@.Calibration.Request.ProcessVariable.WaterContent) ,OTU(@c9c083f8@.Calibration.Request.ProcessVariable.PulseFrequency) ,OTU(@c9c083f8@.Calibration.Request.ProcessVariable.Temperature) ,OTU(@c9c083f8@.Calibration.Request.ProcessVariable.Pressure) ,OTU(@c9c083f8@.Calibration.Request.ProcessVariable.Density) ] ] ,[[XIC(@2dd5c30c@[5].2) [OTL(@c9c083f8@.Calibration.Request.ActionType.ZeroShift) ,COP(@2dd5c30c@[6],@c9c083f8@.Calibration.Request.Value.ZeroShift.Applied,2) ] ,XIO(@2dd5c30c@[5].2) [OTU(@c9c083f8@.Calibration.Request.ActionType.ZeroShift) ,FLL(0,@c9c083f8@.Calibration.Request.Value.ZeroShift.Applied,2) ] ] ,[XIC(@2dd5c30c@[5].3) [OTL(@c9c083f8@.Calibration.Request.ActionType.SetZero) ,COP(@2dd5c30c@[10],@c9c083f8@.Calibration.Request.Value.SetZero.Applied,2) ] ,XIO(@2dd5c30c@[5].3) [OTU(@c9c083f8@.Calibration.Request.ActionType.SetZero) ,FLL(0,@c9c083f8@.Calibration.Request.Value.SetZero.Applied,2) ] ] ,[XIC(@2dd5c30c@[5].4) [OTL(@c9c083f8@.Calibration.Request.ActionType.SetSpan) ,COP(@2dd5c30c@[14],@c9c083f8@.Calibration.Request.Value.SetSpan.Applied,2) ] ,XIO(@2dd5c30c@[5].4) [OTU(@c9c083f8@.Calibration.Request.ActionType.SetSpan) ,FLL(0,@c9c083f8@.Calibration.Request.Value.SetSpan.Applied,2) ] ] ,[XIC(@2dd5c30c@[5].5) [OTL(@c9c083f8@.Calibration.Request.ActionType.SetMid1) ,COP(@2dd5c30c@[18],@c9c083f8@.Calibration.Request.Value.SetMid1.Applied,2) ] ,XIO(@2dd5c30c@[5].5) [OTU(@c9c083f8@.Calibration.Request.ActionType.SetMid1) ,FLL(0,@c9c083f8@.Calibration.Request.Value.SetMid1.Applied,2) ] ] ,[XIC(@2dd5c30c@[5].6) [OTL(@c9c083f8@.Calibration.Request.ActionType.SetMid2) ,COP(@2dd5c30c@[22],@c9c083f8@.Calibration.Request.Value.SetMid2.Applied,2) ] ,XIO(@2dd5c30c@[5].6) [OTU(@c9c083f8@.Calibration.Request.ActionType.SetMid2) ,FLL(0,@c9c083f8@.Calibration.Request.Value.SetMid2.Applied,2) ] ] ,[XIC(@2dd5c30c@[5].7) [OTL(@c9c083f8@.Calibration.Request.ActionType.SetMid3) ,COP(@2dd5c30c@[26],@c9c083f8@.Calibration.Request.Value.SetMid3.Applied,2) ] ,XIO(@2dd5c30c@[5].7) [OTU(@c9c083f8@.Calibration.Request.ActionType.SetMid3) ,FLL(0,@c9c083f8@.Calibration.Request.Value.SetMid3.Applied,2) ] ] ] ] ,EQU(@2dd5c30c@[0],9001) [XIC(@c9c083f8@.Calibration.Response.Trigger) ADD(@c9c083f8@.Calibration.Response.Count,1,@c9c083f8@.Calibration.Response.Count) ,OTU(@c9c083f8@.Calibration.Response.Trigger) ,FLL(0,@5ad51bb9@.Util.Buffer.Calibration[1],6) ] ];
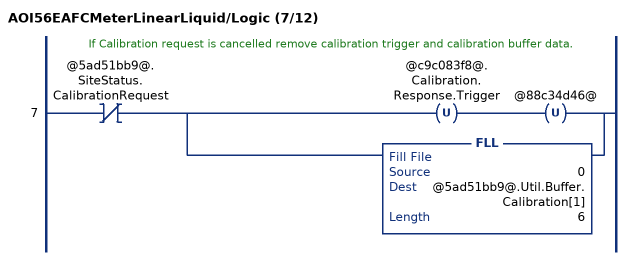
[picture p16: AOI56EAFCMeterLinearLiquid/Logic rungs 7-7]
   // If Calibration request is cancelled remove calibration trigger and calibration buffer data.
   7: XIO(@5ad51bb9@.SiteStatus.CalibrationRequest)[OTU(@c9c083f8@.Calibration.Response.Trigger) OTU(@88c34d46@) ,FLL(0,@5ad51bb9@.Util.Buffer.Calibration[1],6) ];
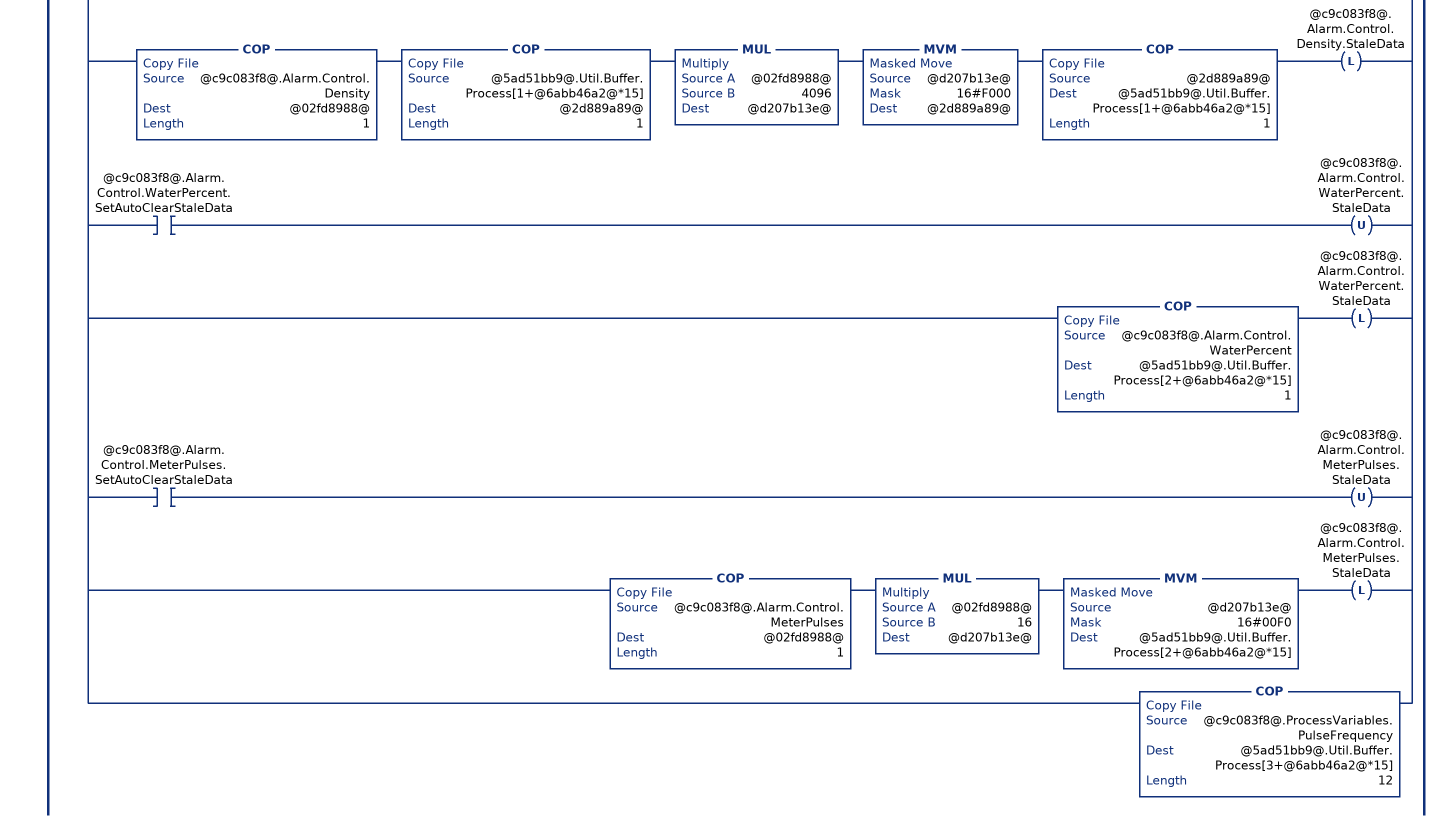
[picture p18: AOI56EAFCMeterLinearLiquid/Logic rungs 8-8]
   // Process variables and process alarms to send to module.
   8: XIC(@012f14ad@)[ADD(16#A000,@d5405e9b@,@b72bc437@) COP(@b72bc437@,@5ad51bb9@.Util.Buffer.Process[@6abb46a2@*15],1) ,[XIC(@c9c083f8@.Alarm.Control.PulseFrequency.SetAutoClearStaleData) OTU(@c9c083f8@.Alarm.Control.PulseFrequency.StaleData) ,COP(@c9c083f8@.Alarm.Control.PulseFrequency,@5ad51bb9@.Util.Buffer.Process[1+@6abb46a2@*15],1) OTL(@c9c083f8@.Alarm.Control.PulseFrequency.StaleData) ] ,[XIC(@c9c083f8@.Alarm.Control.Temperature.SetAutoClearStaleData) OTU(@c9c083f8@.Alarm.Control.Temperature.StaleData) ,COP(@c9c083f8@.Alarm.Control.Temperature,@02fd8988@,1) MUL(@02fd8988@,16,@d207b13e@) MVM(@d207b13e@,16#00F0,@5ad51bb9@.Util.Buffer.Process[1+@6abb46a2@*15]) OTL(@c9c083f8@.Alarm.Control.Temperature.StaleData) ] ,[XIC(@c9c083f8@.Alarm.Control.Pressure.SetAutoClearStaleData) OTU(@c9c083f8@.Alarm.Control.Pressure.StaleData) ,COP(@c9c083f8@.Alarm.Control.Pressure,@02fd8988@,1) MUL(@02fd8988@,256,@d207b13e@) MVM(@d207b13e@,16#0F00,@5ad51bb9@.Util.Buffer.Process[1+@6abb46a2@*15]) OTL(@c9c083f8@.Alarm.Control.Pressure.StaleData) ] ,[XIC(@c9c083f8@.Alarm.Control.Density.SetAutoClearStaleData) OTU(@c9c083f8@.Alarm.Control.Density.StaleData) ,COP(@c9c083f8@.Alarm.Control.Density,@02fd8988@,1) COP(@5ad51bb9@.Util.Buffer.Process[1+@6abb46a2@*15],@2d889a89@,1) MUL(@02fd8988@,4096,@d207b13e@) MVM(@d207b13e@,16#F000,@2d889a89@) COP(@2d889a89@,@5ad51bb9@.Util.Buffer.Process[1+@6abb46a2@*15],1) OTL(@c9c083f8@.Alarm.Control.Density.StaleData) ] ,[XIC(@c9c083f8@.Alarm.Control.WaterPercent.SetAutoClearStaleData) OTU(@c9c083f8@.Alarm.Control.WaterPercent.StaleData) ,COP(@c9c083f8@.Alarm.Control.WaterPercent,@5ad51bb9@.Util.Buffer.Process[2+@6abb46a2@*15],1) OTL(@c9c083f8@.Alarm.Control.WaterPercent.StaleData) ] ,[XIC(@c9c083f8@.Alarm.Control.MeterPulses.SetAutoClearStaleData) OTU(@c9c083f8@.Alarm.Control.MeterPulses.StaleData) ,COP(@c9c083f8@.Alarm.Control.MeterPulses,@02fd8988@,1) MUL(@02fd8988@,16,@d207b13e@) MVM(@d207b13e@,16#00F0,@5ad51bb9@.Util.Buffer.Process[2+@6abb46a2@*15]) OTL(@c9c083f8@.Alarm.Control.MeterPulses.StaleData) ] ,COP(@c9c083f8@.ProcessVariables.PulseFrequency,@5ad51bb9@.Util.Buffer.Process[3+@6abb46a2@*15],12) ];
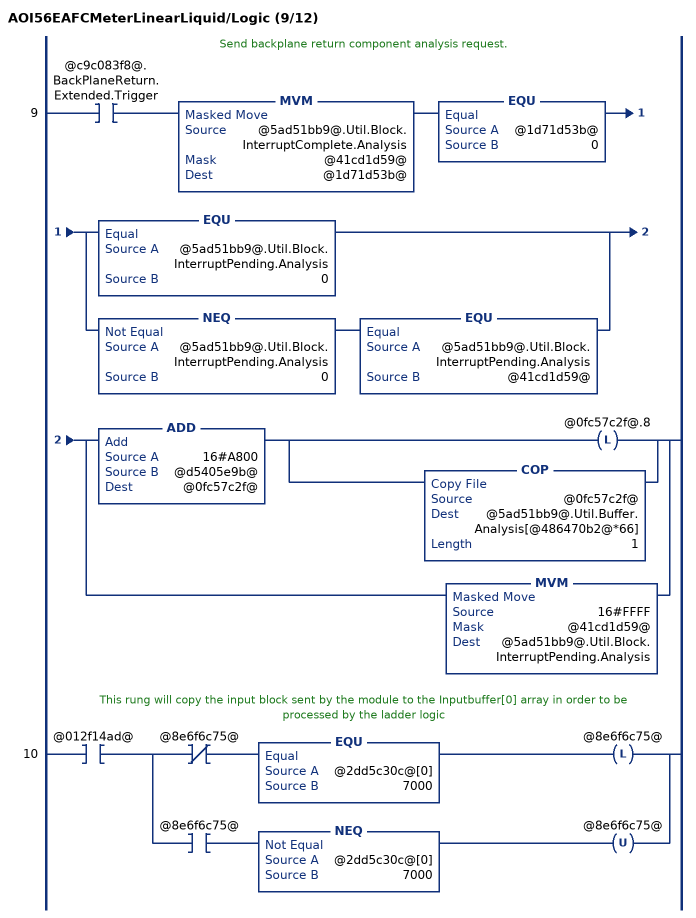
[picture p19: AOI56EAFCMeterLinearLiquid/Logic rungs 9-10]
   // Send backplane return component analysis request.
   9: XIC(@c9c083f8@.BackPlaneReturn.Extended.Trigger)MVM(@5ad51bb9@.Util.Block.InterruptComplete.Analysis,@41cd1d59@,@1d71d53b@)EQU(@1d71d53b@,0)[EQU(@5ad51bb9@.Util.Block.InterruptPending.Analysis,0) ,NEQ(@5ad51bb9@.Util.Block.InterruptPending.Analysis,0) EQU(@5ad51bb9@.Util.Block.InterruptPending.Analysis,@41cd1d59@) ][ADD(16#A800,@d5405e9b@,@0fc57c2f@) [OTL(@0fc57c2f@.8) ,COP(@0fc57c2f@,@5ad51bb9@.Util.Buffer.Analysis[@486470b2@*66],1) ] ,MVM(16#FFFF,@41cd1d59@,@5ad51bb9@.Util.Block.InterruptPending.Analysis) ];
   // This rung will copy the input block sent by the module to the Inputbuffer[0] array in order to be processed by the ladder logic
   10: XIC(@012f14ad@)[XIO(@8e6f6c75@) EQU(@2dd5c30c@[0],7000) OTL(@8e6f6c75@) ,XIC(@8e6f6c75@) NEQ(@2dd5c30c@[0],7000) OTU(@8e6f6c75@) ];
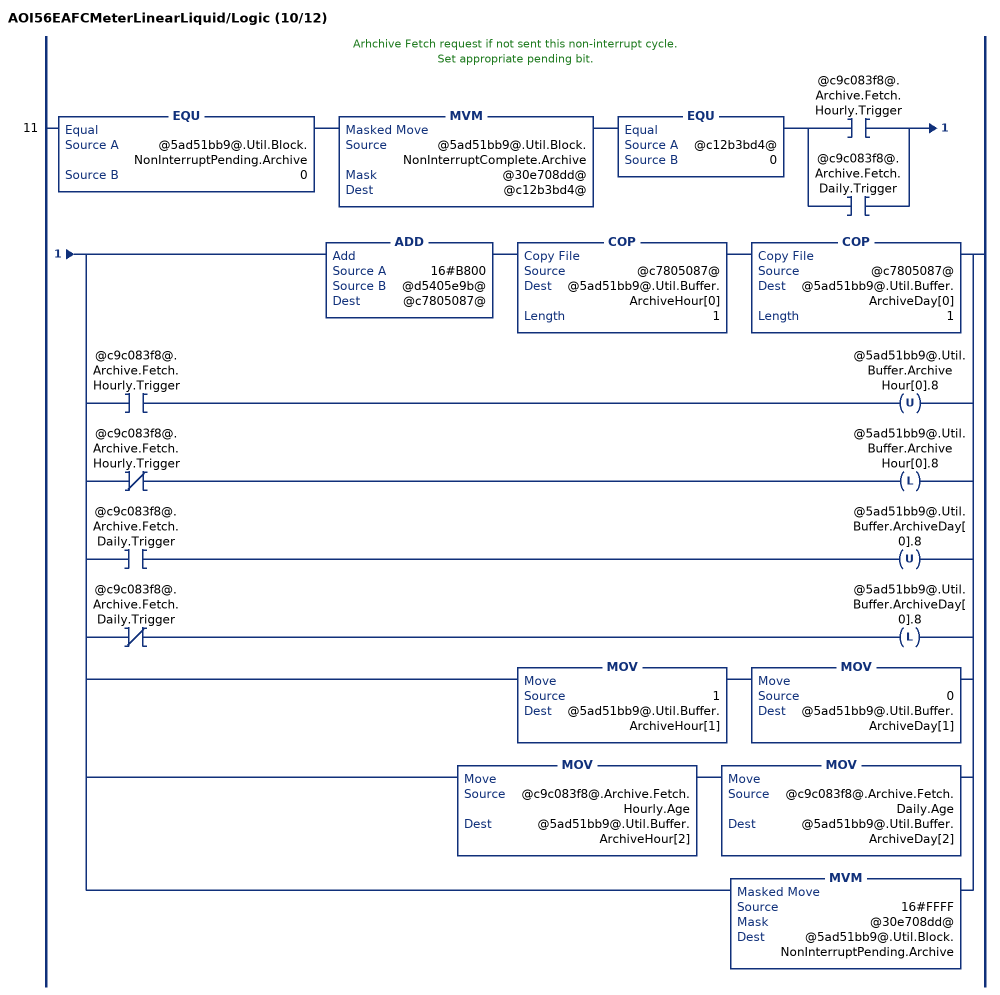
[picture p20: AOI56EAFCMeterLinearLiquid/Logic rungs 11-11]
   // Arhchive Fetch request if not sent this non-interrupt cycle.
   // Set appropriate pending bit.
   11: EQU(@5ad51bb9@.Util.Block.NonInterruptPending.Archive,0)MVM(@5ad51bb9@.Util.Block.NonInterruptComplete.Archive,@30e708dd@,@c12b3bd4@)EQU(@c12b3bd4@,0)[XIC(@c9c083f8@.Archive.Fetch.Hourly.Trigger) ,XIC(@c9c083f8@.Archive.Fetch.Daily.Trigger) ][ADD(16#B800,@d5405e9b@,@c7805087@) COP(@c7805087@,@5ad51bb9@.Util.Buffer.ArchiveHour[0],1) COP(@c7805087@,@5ad51bb9@.Util.Buffer.ArchiveDay[0],1) ,[XIC(@c9c083f8@.Archive.Fetch.Hourly.Trigger) OTU(@5ad51bb9@.Util.Buffer.ArchiveHour[0].8) ,XIO(@c9c083f8@.Archive.Fetch.Hourly.Trigger) OTL(@5ad51bb9@.Util.Buffer.ArchiveHour[0].8) ] ,[XIC(@c9c083f8@.Archive.Fetch.Daily.Trigger) OTU(@5ad51bb9@.Util.Buffer.ArchiveDay[0].8) ,XIO(@c9c083f8@.Archive.Fetch.Daily.Trigger) OTL(@5ad51bb9@.Util.Buffer.ArchiveDay[0].8) ] ,MOV(1,@5ad51bb9@.Util.Buffer.ArchiveHour[1]) MOV(0,@5ad51bb9@.Util.Buffer.ArchiveDay[1]) ,MOV(@c9c083f8@.Archive.Fetch.Hourly.Age,@5ad51bb9@.Util.Buffer.ArchiveHour[2]) MOV(@c9c083f8@.Archive.Fetch.Daily.Age,@5ad51bb9@.Util.Buffer.ArchiveDay[2]) ,MVM(16#FFFF,@30e708dd@,@5ad51bb9@.Util.Block.NonInterruptPending.Archive) ];
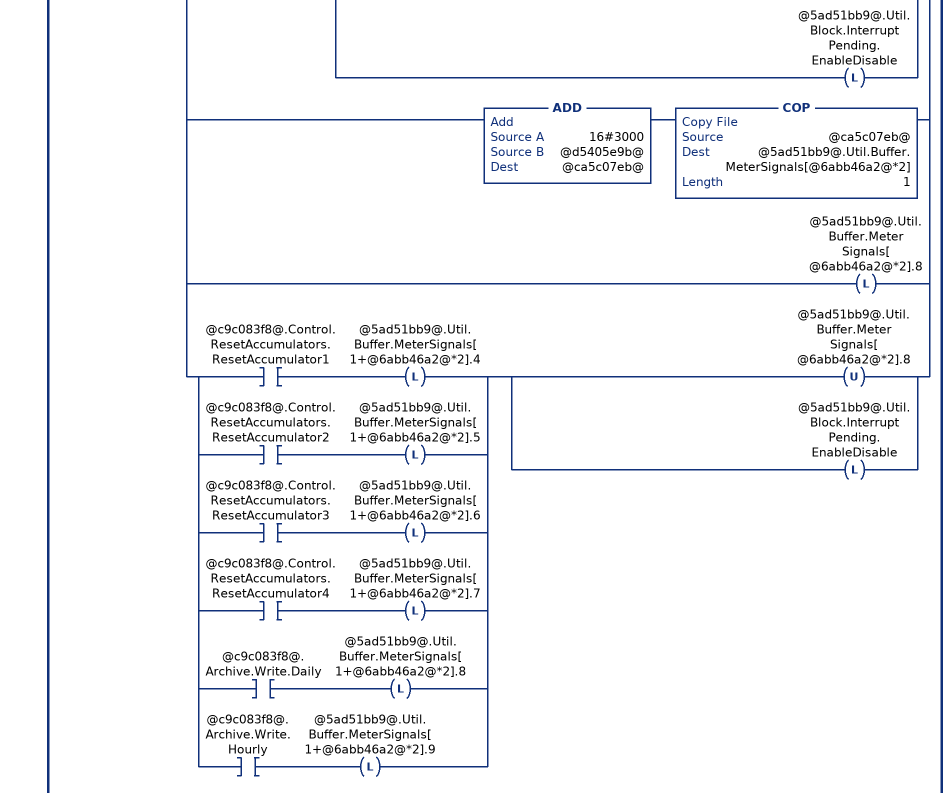
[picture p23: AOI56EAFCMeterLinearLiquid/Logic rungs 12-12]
   // Meter Enable.
   // Meter Disable.
   // Stream Select.
   // Stream Enable.
   // Stream Disable.
   // Set pending bit if not set this interrupt cycle.
   12: XIO(@5ad51bb9@.Util.Block.InterruptComplete.EnableDisable)[LIM(1,@c9c083f8@.Control.Stream.Selected,16) CPT(@2c793ec3@,2**(@c9c083f8@.Control.Stream.Selected-1)) ,[XIC(@c9c083f8@.Control.Meter.Enable) MVM(16#FFFF,@30e708dd@,@5ad51bb9@.Util.Buffer.MeterEnableDisable[1]) MVM(16#0000,@30e708dd@,@5ad51bb9@.Util.Buffer.MeterEnableDisable[3]) ,XIC(@c9c083f8@.Control.Meter.Disable) MVM(16#FFFF,@30e708dd@,@5ad51bb9@.Util.Buffer.MeterEnableDisable[3]) MVM(16#0000,@30e708dd@,@5ad51bb9@.Util.Buffer.MeterEnableDisable[1]) ] OTL(@5ad51bb9@.Util.Block.InterruptPending.EnableDisable) ,[ADD(16#CC00,@d5405e9b@,@c591a840@) COP(@c591a840@,@5ad51bb9@.Util.Buffer.StreamEnable[@6abb46a2@*3],1) ,XIO(@c9c083f8@.Control.Stream.EnableSelected) OTL(@5ad51bb9@.Util.Buffer.StreamEnable[@6abb46a2@*3].8) ,XIC(@c9c083f8@.Control.Stream.EnableSelected) [OTU(@5ad51bb9@.Util.Buffer.StreamEnable[@6abb46a2@*3].8) ,COP(@2c793ec3@,@5ad51bb9@.Util.Buffer.StreamEnable[1+@6abb46a2@*3],1) ,OTL(@5ad51bb9@.Util.Block.InterruptPending.EnableDisable) ] ] ,[ADD(16#C800,@d5405e9b@,@ba4ec91a@) COP(@ba4ec91a@,@5ad51bb9@.Util.Buffer.StreamDisable[@6abb46a2@*3],1) ,XIO(@c9c083f8@.Control.Stream.DisableSelected) OTL(@5ad51bb9@.Util.Buffer.StreamDisable[@6abb46a2@*3].8) ,XIC(@c9c083f8@.Control.Stream.DisableSelected) [OTU(@5ad51bb9@.Util.Buffer.StreamDisable[@6abb46a2@*3].8) ,COP(@2c793ec3@,@5ad51bb9@.Util.Buffer.StreamDisable[1+@6abb46a2@*3],1) ,OTL(@5ad51bb9@.Util.Block.InterruptPending.EnableDisable) ] ] ,[ADD(16#3C00,@d5405e9b@,@268d238f@) COP(@268d238f@,@5ad51bb9@.Util.Buffer.StreamSelect[@6abb46a2@*2],1) ,XIO(@c9c083f8@.Control.Stream.SetSelectedToActive) OTL(@5ad51bb9@.Util.Buffer.StreamSelect[@6abb46a2@*2].8) ,XIC(@c9c083f8@.Control.Stream.SetSelectedToActive) [OTU(@5ad51bb9@.Util.Buffer.StreamSelect[@6abb46a2@*2].8) ,MOV(@c9c083f8@.Control.Stream.Selected,@5ad51bb9@.Util.Buffer.StreamSelect[1+@6abb46a2@*2]) ,OTL(@5ad51bb9@.Util.Block.InterruptPending.EnableDisable) ] ] ,[ADD(16#3000,@d5405e9b@,@ca5c07eb@) COP(@ca5c07eb@,@5ad51bb9@.Util.Buffer.MeterSignals[@6abb46a2@*2],1) ,OTL(@5ad51bb9@.Util.Buffer.MeterSignals[@6abb46a2@*2].8) ,[XIC(@c9c083f8@.Control.ResetAccumulators.ResetAccumulator1) OTL(@5ad51bb9@.Util.Buffer.MeterSignals[1+@6abb46a2@*2].4) ,XIC(@c9c083f8@.Control.ResetAccumulators.ResetAccumulator2) OTL(@5ad51bb9@.Util.Buffer.MeterSignals[1+@6abb46a2@*2].5) ,XIC(@c9c083f8@.Control.ResetAccumulators.ResetAccumulator3) OTL(@5ad51bb9@.Util.Buffer.MeterSignals[1+@6abb46a2@*2].6) ,XIC(@c9c083f8@.Control.ResetAccumulators.ResetAccumulator4) OTL(@5ad51bb9@.Util.Buffer.MeterSignals[1+@6abb46a2@*2].7) ,XIC(@c9c083f8@.Archive.Write.Daily) OTL(@5ad51bb9@.Util.Buffer.MeterSignals[1+@6abb46a2@*2].8) ,XIC(@c9c083f8@.Archive.Write.Hourly) OTL(@5ad51bb9@.Util.Buffer.MeterSignals[1+@6abb46a2@*2].9) ] [OTU(@5ad51bb9@.Util.Buffer.MeterSignals[@6abb46a2@*2].8) ,OTL(@5ad51bb9@.Util.Block.InterruptPending.EnableDisable) ] ] ];
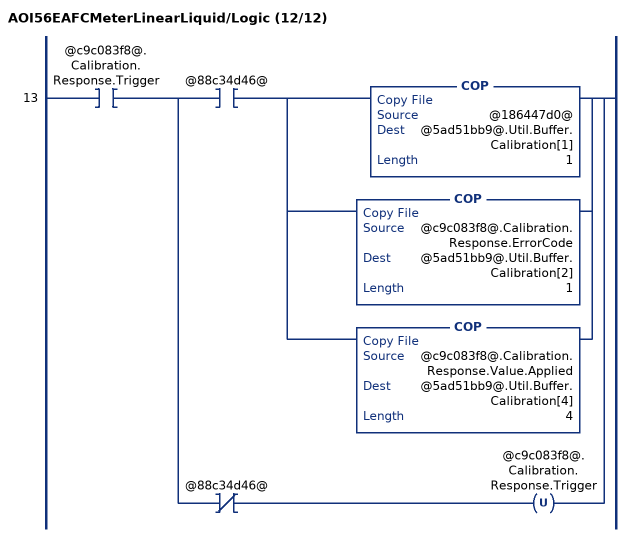
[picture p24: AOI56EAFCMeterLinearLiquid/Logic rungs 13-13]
   13: XIC(@c9c083f8@.Calibration.Response.Trigger)[XIC(@88c34d46@) [COP(@186447d0@,@5ad51bb9@.Util.Buffer.Calibration[1],1) ,COP(@c9c083f8@.Calibration.Response.ErrorCode,@5ad51bb9@.Util.Buffer.Calibration[2],1) ,COP(@c9c083f8@.Calibration.Response.Value.Applied,@5ad51bb9@.Util.Buffer.Calibration[4],4) ] ,XIO(@88c34d46@) OTU(@c9c083f8@.Calibration.Response.Trigger) ];
END_ROUTINE

ROUTINE Prescan   (* ladder *)
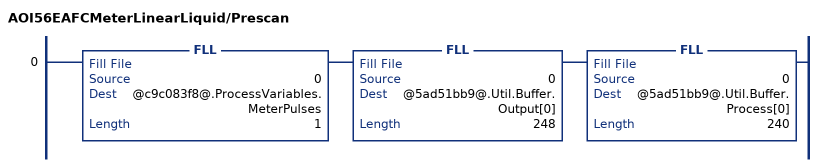
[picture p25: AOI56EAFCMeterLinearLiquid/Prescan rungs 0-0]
   0: FLL(0,@c9c083f8@.ProcessVariables.MeterPulses,1)FLL(0,@5ad51bb9@.Util.Buffer.Output[0],248)FLL(0,@5ad51bb9@.Util.Buffer.Process[0],240);
END_ROUTINE
END_ADD_ON_INSTRUCTION

VAR_GLOBAL   (* controller tags *)
   AFC : AFCEModuleDef;
   Local:1:I : AB:1756_MODULE_INT_500Bytes:I:0;
   AOI56EAFCMeter04LinearLiquid : AOI56EAFCMeterLinearLiquid;
   AFCMeter04LinearLiquid : AFCEMeterLinearLiquid;
END_VAR

PROGRAM MainProgram

ROUTINE MainRoutine   (* ladder *)
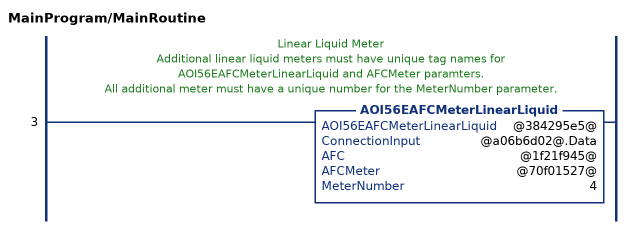
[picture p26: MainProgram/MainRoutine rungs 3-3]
   // Linear Liquid Meter
   // Additional linear liquid meters must have unique tag names for AOI56EAFCMeterLinearLiquid and AFCMeter paramters.
   // All additional meter must have a unique number for the MeterNumber parameter.
   3: AOI56EAFCMeterLinearLiquid(@384295e5@,@a06b6d02@.Data,@1f21f945@,@70f01527@,4);
END_ROUTINE
END_PROGRAM
